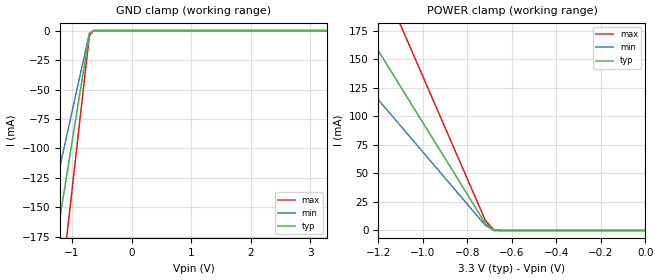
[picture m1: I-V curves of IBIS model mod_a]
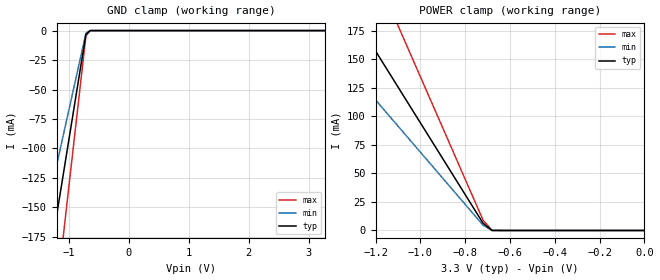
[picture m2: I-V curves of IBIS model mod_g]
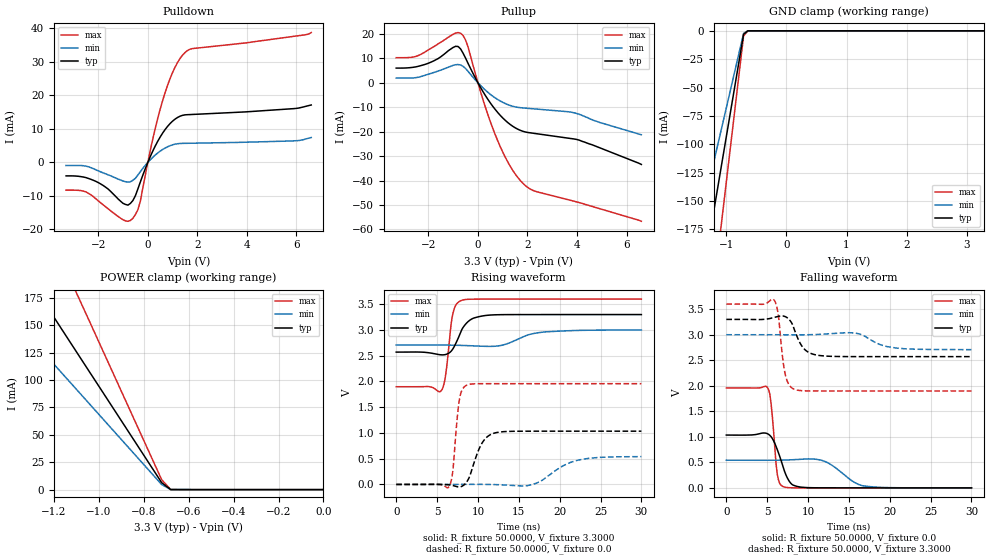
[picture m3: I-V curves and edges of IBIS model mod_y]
| IBIS (I/O, Buffer, Information, Specification) Model, officially
| electronic behavioral standard for Buffer structures of digital pins.
[IBIS ver]  4.0
[File name] 54hc138_3v3_rev1.ibs
[File Rev]  1.0
[Date]   12 Feb 2019
[Source]   CAD & Design Services (Catania) - STMicroelectronics
[Notes]
  (Note1) This IBIS model is the model of the product with package
   (Flat16 package elements);
  (Note2) This IBIS model is extracted with nominal 3.3V power supply
   (min:3.0V, typ:3.3V, max:3.6V);
  (Note3) This model has few Warnings about the non-monotonicity
   of I-V curves, but they are not indicative of problems
   inside the model;
[Disclaimer]
   Customers are solely responsible for all aspects of their
   own product designs or applications using this IBIS Model.
   STMicroelectronics assumes no liability for Custmer Designs
   and applications associated to this IBIS Model.
   In the use of this IBIS Model Customer shall not modify,
   disassemble, alter this Model in whole or in part.
   If Customers do not accept these terms, the IBIS Model
   may not be used. For any problems or modifications please
   contact STMicroelectronics (www.st.com).
[Copyright] (c) 2019 STMicroelectronics
|   Component 54HC138
[Component] 54HC138
[Manufacturer] STMicroelectronics
[Package]
| variable  typ   min   max
R_pkg   0.0   0.0   0.0
L_pkg   0.0H   0.0H   0.0H
C_pkg   0.0F   0.0F   0.0F
[Pin]   signal_name   model_name   R_pin   L_pin   C_pin
1   A   mod_a   87.8m   2.68nH   1.16pF
2   B   mod_a   53.6m   1.94nH   1.11pF
3   C   mod_a   34.1m   1.02nH   0.87pF
4   G2AN   mod_g   34.1m   1.02nH   0.87pF
5   G2BN   mod_g   34.1m   1.02nH   0.87pF
6   G1   mod_g   34.1m   1.02nH   0.87pF
7   Y7N   mod_y   53.6m   1.94nH   1.11pF
8   VSS   GND   87.8m   2.68nH   1.16pF
9   Y6N   mod_y   87.8m   2.68nH   1.16pF
10   Y5N   mod_y   53.6m   1.94nH   1.11pF
11   Y4N   mod_y   34.1m   1.02nH   0.87pF
12   Y3N   mod_y   34.1m   1.02nH   0.87pF
13   Y2N   mod_y   34.1m   1.02nH   0.87pF
14   Y1N   mod_y   34.1m   1.02nH   0.87pF
15   Y0N   mod_y   53.6m   1.94nH   1.11pF
16   VDD   POWER   87.8m   2.68nH   1.16pF
| Models and submodels in the file (3): mod_a (Input), mod_g (Input), mod_y (I/O)
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|   Model mod_a
[Model]   mod_a
Model_type  Input
Vinl   =   1.000V
Vinh   =   2.200V
C_comp   1.112pF   1.062pF   1.164pF
[Temperature Range]  25.0000   0.1250k   -55.0000
[Voltage Range]   3.3000V   3.0000V   3.6000V
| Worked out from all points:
|   GND clamp passes 1 mA (typ) near -0.66 V on its own axis
|   POWER clamp passes 1 mA (typ) near -0.69 V on its own axis
[GND_clamp]
|Voltage   I(typ)   I(min)   I(max)
-3.3V     -815.7mA   -595.5mA   -1.169A
-1.48V    -245.6mA   -178.6mA   -350.7mA
-1.41V    -223.5mA   -162.6mA   -319.2mA
-1.27V    -179.5mA   -130.5mA   -256.3mA
-1.2V     -157.4mA   -114.5mA   -224.8mA
-1.13V    -135.4mA   -98.48mA   -193.3mA
-1.06V    -113.3mA   -82.45mA   -161.9mA
-710mV    -3.148mA   -2.29mA    -4.496mA
-640mV    -12.11uA   -11.04uA   -87.08uA
3.28V     8.59nA     6.387nA    13.14nA
[POWER_clamp]
|Voltage   I(typ)   I(min)   I(max)
-3.28V    812.3mA    590.9mA    1.16A
-1.48V    245.6mA    178.6mA    350.7mA
-1.44V    233mA      169.5mA    332.7mA
-1.28V    182.6mA    132.8mA    260.8mA
-1.24V    170mA      123.7mA    242.8mA
-1.12V    132.2mA    96.19mA    188.8mA
-1.08V    119.6mA    87.03mA    170.8mA
-720mV    6.297mA    4.581mA    8.992mA
-680mV    2.835uA    981.2nA    118uA
0V        0A         0A         0A
|   Model mod_g
[Model]   mod_g
Model_type  Input
Vinl   =   1.000V
Vinh   =   2.200V
C_comp   0.925pF   0.883pF   0.968pF
[Temperature Range]  25.0000   0.1250k   -55.0000
[Voltage Range]   3.3000V   3.0000V   3.6000V
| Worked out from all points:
|   GND clamp passes 1 mA (typ) near -0.66 V on its own axis
|   POWER clamp passes 1 mA (typ) near -0.69 V on its own axis
[GND_clamp]
|Voltage   I(typ)   I(min)   I(max)
-3.3V     -815.7mA   -595.5mA   -1.169A
-1.48V    -245.6mA   -178.6mA   -350.7mA
-1.41V    -223.5mA   -162.6mA   -319.2mA
-1.27V    -179.5mA   -130.5mA   -256.3mA
-1.2V     -157.4mA   -114.5mA   -224.8mA
-1.13V    -135.4mA   -98.48mA   -193.3mA
-1.06V    -113.3mA   -82.45mA   -161.9mA
-710mV    -3.148mA   -2.29mA    -4.496mA
-640mV    -12.11uA   -11.04uA   -87.08uA
3.28V     8.59nA     6.387nA    13.14nA
[POWER_clamp]
|Voltage   I(typ)   I(min)   I(max)
-3.28V    812.3mA    590.9mA    1.16A
-1.48V    245.6mA    178.6mA    350.7mA
-1.44V    233mA      169.5mA    332.7mA
-1.28V    182.6mA    132.8mA    260.8mA
-1.24V    170mA      123.7mA    242.8mA
-1.12V    132.2mA    96.19mA    188.8mA
-1.08V    119.6mA    87.03mA    170.8mA
-720mV    6.297mA    4.581mA    8.992mA
-680mV    2.835uA    981.2nA    118uA
0V        0A         0A         0A
|   Model mod_y
[Model]   mod_y
Model_type I/O
Polarity   Non-Inverting
Vinl   =   0.800V
Vinh   =   1.220V
Vmeas  =   1.650V
Cref   =   50pF
C_comp   2.668pF   2.433pF   2.793pF
[Temperature Range]  25.0000   0.1250k   -55.0000
[Voltage Range]   3.3000V   3.0000V   3.6000V
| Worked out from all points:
|   slope of the pulldown table from 0 to 0.495 V, typ, clamps not added: 65.8 ohm
|   slope of the pullup table from 0 to 0.495 V, typ, clamps not added: 60.6 ohm
|   GND clamp passes 1 mA (typ) near -0.66 V on its own axis
|   POWER clamp passes 1 mA (typ) near -0.69 V on its own axis
|   rising waveform, R_fixture 50.0000, V_fixture 3.3000: 20-80 % time 1.52ns typ, 3.06ns min, 720ps max; typ from 2.57 V to 3.3 V
|   rising waveform, R_fixture 50.0000, V_fixture 0.0: 20-80 % time 1.5ns typ, 3.32ns min, 649ps max; typ from 0 V to 1.03 V
|   falling waveform, R_fixture 50.0000, V_fixture 0.0: 20-80 % time 1.38ns typ, 2.67ns min, 615ps max; typ from 1.03 V to 0 V
|   falling waveform, R_fixture 50.0000, V_fixture 3.3000: 20-80 % time 1.35ns typ, 2.48ns min, 738ps max; typ from 3.3 V to 2.57 V
[Pulldown]
|Voltage   I(typ)   I(min)   I(max)
-3.3V     -4.012mA   -917uA     -8.265mA
-2.5V     -4.523mA   -1.114mA   -8.791mA
-1.8V     -6.888mA   -3.138mA   -12.65mA
-1V       -12.21mA   -5.547mA   -17.1mA
-700mV    -12.21mA   -5.761mA   -17.3mA
-400mV    -7.89mA    -3.758mA   -14.12mA
-300mV    -5.803mA   -2.74mA    -11.52mA
200mV     3.377mA    1.528mA    6.954mA
700mV     9.821mA    4.303mA    20.86mA
1.1V      12.92mA    5.447mA    28.41mA
1.5V      14.19mA    5.697mA    32.77mA
6.6V      17.14mA    7.443mA    38.74mA
[Pullup]
|Voltage   I(typ)   I(min)   I(max)
-3.3V     6.012mA    1.917mA    10.27mA
-2.5V     6.523mA    2.114mA    10.79mA
-900mV    14.93mA    7.387mA    20.32mA
-700mV    13.85mA    7.279mA    20.26mA
-400mV    7.973mA    4.698mA    14.71mA
200mV     -3.547mA   -2.058mA   -6.767mA
800mV     -12.17mA   -6.856mA   -23.74mA
1.3V      -17.03mA   -9.277mA   -34.08mA
1.8V      -19.79mA   -10.27mA   -40.94mA
2.3V      -20.74mA   -10.7mA    -44.35mA
4V        -23.21mA   -12.6mA    -48.77mA
6.6V      -33.41mA   -21.27mA   -56.67mA
[GND_clamp]
|Voltage   I(typ)   I(min)   I(max)
-3.3V     -815.7mA   -595.5mA   -1.169A
-1.48V    -245.6mA   -178.6mA   -350.7mA
-1.41V    -223.5mA   -162.6mA   -319.2mA
-1.27V    -179.5mA   -130.5mA   -256.3mA
-1.2V     -157.4mA   -114.5mA   -224.8mA
-1.13V    -135.4mA   -98.48mA   -193.3mA
-1.06V    -113.3mA   -82.45mA   -161.9mA
-710mV    -3.148mA   -2.29mA    -4.496mA
-640mV    -12.11uA   -11.04uA   -87.08uA
3.28V     8.59nA     6.387nA    13.14nA
[POWER_clamp]
|Voltage   I(typ)   I(min)   I(max)
-3.28V    812.3mA    590.9mA    1.16A
-1.48V    245.6mA    178.6mA    350.7mA
-1.44V    233mA      169.5mA    332.7mA
-1.28V    182.6mA    132.8mA    260.8mA
-1.24V    170mA      123.7mA    242.8mA
-1.12V    132.2mA    96.19mA    188.8mA
-1.08V    119.6mA    87.03mA    170.8mA
-720mV    6.297mA    4.581mA    8.992mA
-680mV    2.835uA    981.2nA    118uA
0V        0A         0A         0A
[Ramp]
| variable   typ   min   max
dV/dt_r   0.6205/1.5500n   0.6486/1.9432n   1.1745/0.6726n
dV/dt_f   0.4376/1.4371n   0.9400/2.6767n   1.0212/0.7932n
R_load = 50.0000
[Rising Waveform]
R_fixture= 50.0000
V_fixture= 3.3000
V_fixture_min= 3.0000
V_fixture_max= 3.6000
|time   V(typ)   V(min)   V(max)
0s        2.571V     2.707V     1.898V
5.575ns   2.517V     2.708V     1.833V
6.025ns   2.523V     2.707V     2.101V
6.925ns   2.631V     2.705V     3.311V
7.325ns   2.751V     2.704V     3.493V
8.025ns   3.006V     2.701V     3.577V
9.225ns   3.213V     2.694V     3.599V
11.37ns   3.289V     2.682V     3.6V
17.75ns   3.3V       2.955V     3.6V
30ns      3.3V       3V         3.6V
[Rising Waveform]
R_fixture= 50.0000
V_fixture= 0.0
V_fixture_min= 0.0
V_fixture_max= 0.0
|time   V(typ)   V(min)   V(max)
0s        0V         0V         0V
6.5ns     -9.231mV   488.4uV    -35.8mV
6.95ns    -22.73mV   653.9uV    294.1mV
7.75ns    -50.13mV   907.1uV    1.665V
8.65ns    54.63mV    1.104mV    1.93V
10.35ns   759.7mV    1.048mV    1.957V
11.95ns   994.5mV    -2.355mV   1.958V
16.72ns   1.034V     1.144mV    1.958V
22.35ns   1.035V     475.6mV    1.958V
30ns      1.035V     540.8mV    1.958V
[Falling Waveform]
R_fixture= 50.0000
V_fixture= 0.0
V_fixture_min= 0.0
V_fixture_max= 0.0
|time   V(typ)   V(min)   V(max)
0s        1.034V     541.6mV    1.958V
5.025ns   1.061V     540.7mV    1.968V
5.475ns   1.003V     541mV      1.655V
6.225ns   753.9mV    541.8mV    279.2mV
6.975ns   397.7mV    543.9mV    22.45mV
7.875ns   92.52mV    549.2mV    2.254mV
9.175ns   13.37mV    560.5mV    155.6uV
12.1ns    510.9uV    514.5mV    658.4nV
16.77ns   7.706uV    38.44mV    -57.02nV
30ns      -44.01nV   25.26uV    -57.18nV
[Falling Waveform]
R_fixture= 50.0000
V_fixture= 3.3000
V_fixture_min= 3.0000
V_fixture_max= 3.6000
|time   V(typ)   V(min)   V(max)
0s        3.3V       3V         3.6V
5.9ns     3.341V     3V         3.669V
6.4ns     3.36V      3V         3.343V
7.2ns     3.355V     2.999V     2.231V
8.35ns    3.089V     2.999V     1.929V
9.5ns     2.726V     2.999V     1.902V
11.3ns    2.595V     3.006V     1.898V
15.97ns   2.571V     3.026V     1.898V
20.85ns   2.571V     2.738V     1.898V
30ns      2.571V     2.708V     1.898V
